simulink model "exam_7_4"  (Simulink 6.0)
settings: Solver=VariableStepDiscrete  StartTime=0.0  StopTime=10.0  RelTol=1e-3

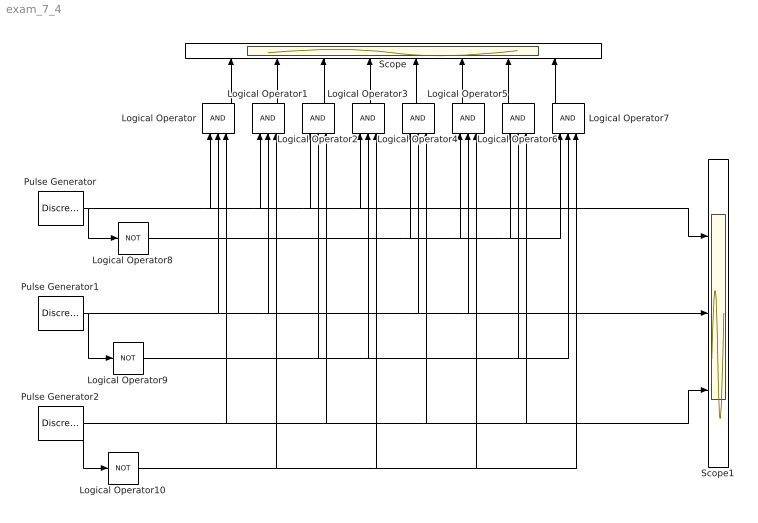
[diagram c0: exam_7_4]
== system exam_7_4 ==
  Logical Operator{,1..7} (8 alike) : Logic  Orientation=up  Inputs=3  AllPortsSameDT=off  OutDataTypeMode=Boolean
  Logical Operator10 : Logic  Operator=NOT  AllPortsSameDT=off  OutDataTypeMode=Boolean
  Logical Operator8 : Logic  Operator=NOT  AllPortsSameDT=off  OutDataTypeMode=Boolean
  Logical Operator9 : Logic  Operator=NOT  AllPortsSameDT=off  OutDataTypeMode=Boolean
  Pulse Generator : DiscretePulseGenerator  Amplitude=2  PhaseDelay=1
  Pulse Generator1 : DiscretePulseGenerator  Amplitude=2  PhaseDelay=1  SampleTime=2
  Pulse Generator2 : DiscretePulseGenerator  Amplitude=2  PhaseDelay=1  SampleTime=4
  Scope : Scope  NumInputPorts=8
  Scope1 : Scope  NumInputPorts=3
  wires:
  Pulse Generator/1 -> Logical Operator8/1, Logical Operator/1, Logical Operator1/1, Logical Operator2/1, Scope1/1, Logical Operator3/1
  Pulse Generator1/1 -> Logical Operator9/1, Logical Operator/2, Logical Operator1/2, Logical Operator4/2, Scope1/2, Logical Operator5/2
  Pulse Generator2/1 -> Logical Operator10/1, Logical Operator/3, Logical Operator2/3, Logical Operator4/3, Scope1/3, Logical Operator6/3
  Logical Operator/1 -> Scope/1
  Logical Operator1/1 -> Scope/2
  Logical Operator2/1 -> Scope/3
  Logical Operator3/1 -> Scope/4
  Logical Operator4/1 -> Scope/5
  Logical Operator5/1 -> Scope/6
  Logical Operator6/1 -> Scope/7
  Logical Operator7/1 -> Scope/8
  Logical Operator8/1 -> Logical Operator7/1, Logical Operator6/1, Logical Operator5/1, Logical Operator4/1
  Logical Operator9/1 -> Logical Operator2/2, Logical Operator3/2, Logical Operator7/2, Logical Operator6/2
  Logical Operator10/1 -> Logical Operator1/3, Logical Operator3/3, Logical Operator7/3, Logical Operator5/3
